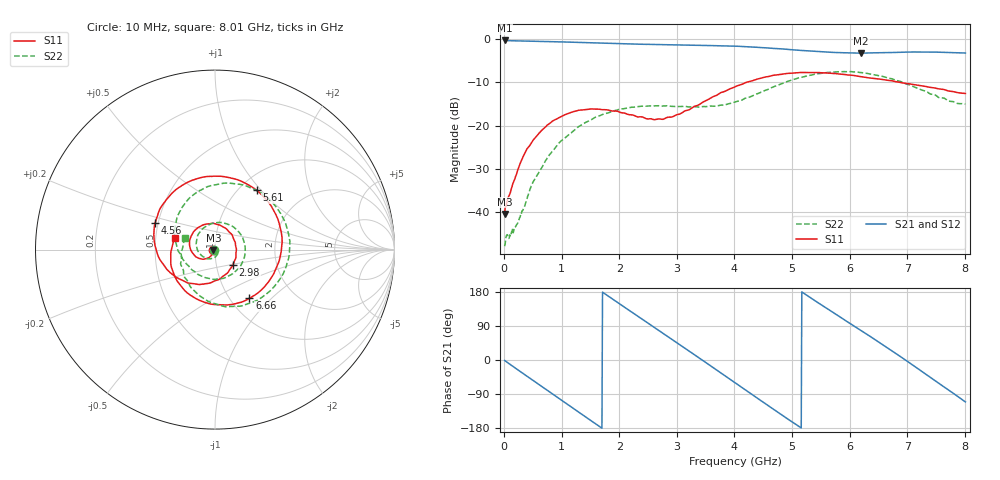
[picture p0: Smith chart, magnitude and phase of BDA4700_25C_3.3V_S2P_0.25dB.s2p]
!Agilent Technologies,E5071B,MY42404982,A.09.10
!Date: Mon Oct 20 18:03:04 2025
!Data & Calibration Information:
!Freq	S11:SOLT2(ON)	S21:SOLT2(ON)	S12:SOLT2(ON)	S22:SOLT2(ON)
# Hz S RI R 50
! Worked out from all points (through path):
!   801 points, 10 MHz to 8.01 GHz, reference 50 ohm
!   highest |S21| = -0.37 dB at 10 MHz (marker M1); lowest = -3.3 dB at 6.2 GHz (marker M2)
!   group delay of S21, straight-line fit = 286 ps
!   lowest |S11| = -40.4 dB at 10 MHz (marker M3), VSWR 1.02, Z = 49.1 - j0.238 ohm
!   |S11| at or under -10 dB: start of sweep to 4.215 GHz; 6.86 GHz to end of sweep
!   |S22| runs from -47.8 to -7.5 dB; largest |S21 - S12| = 0.011
!   S11 on the Smith chart (normalised r, x): 10 MHz: 0.98, -0.00; 2.98 GHz: 1.20, -0.21; 4.56 GHz: 0.48, +0.16; 5.61 GHz: 1.19, +0.95; 6.66 GHz: 1.22, -0.75; 8.01 GHz: 0.63, +0.09
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1e7  -0.00927 -0.00243  0.9577 -0.0205  0.9574 -0.0212  -0.00405 -0.000447
3.6e8  -0.0273 -0.0393  0.7354 -0.5892  0.735 -0.5896  0.0118 -0.000516
7.1e8  -0.0803 -0.0511  0.2291 -0.903  0.2287 -0.903  0.00503 -0.0378
1.02e9  -0.1289 -0.0133  -0.2922 -0.8734  -0.2922 -0.873  -0.0482 -0.049
1.35e9  -0.1377 0.0624  -0.7279 -0.5431  -0.7278 -0.5434  -0.1014 0.0106
1.64e9  -0.0935 0.1233  -0.89 -0.0992  -0.8904 -0.0987  -0.0859 0.0957
1.92e9  -0.021 0.1456  -0.8139 0.3439  -0.8145 0.3435  -0.00336 0.1485
2.32e9  0.0793 0.0975  -0.3781 0.7821  -0.3783 0.7821  0.1337 0.0972
2.68e9  0.1191 0.00486  0.1689 0.8426  0.168 0.8425  0.1643 -0.0414
2.98e9  0.0998 -0.0861  0.5733 0.6297  0.5724 0.6289  0.0986 -0.1343
3.48e9  -0.0337 -0.1877  0.8378 -0.063  0.8381 -0.063  -0.0666 -0.1517
4.01e9  -0.2486 -0.1294  0.4128 -0.7114  0.4143 -0.7102  -0.1786 -0.0541
4.56e9  -0.3335 0.1484  -0.3652 -0.6964  -0.3645 -0.6977  -0.2207 0.1333
4.95e9  -0.1951 0.3494  -0.6987 -0.2804  -0.6987 -0.2845  -0.1231 0.3031
5.35e9  0.0655 0.4036  -0.6825 0.2308  -0.684 0.2269  0.1153 0.3659
5.61e9  0.2317 0.3317  -0.5017 0.4912  -0.5031 0.4914  0.2797 0.2986
6.2e9  0.3645 -0.034  0.1428 0.6687  0.1522 0.6698  0.3987 -0.0867
6.66e9  0.1915 -0.2717  0.5911 0.3636  0.5924 0.3629  0.1901 -0.2998
6.68e9  0.1804 -0.278  0.6033 0.3436  0.6055 0.3421  0.1782 -0.3035
7.24e9  -0.1375 -0.2536  0.6199 -0.3387  0.6188 -0.3386  -0.111 -0.2338
7.63e9  -0.2445 -0.0917  0.2383 -0.6565  0.2379 -0.6567  -0.1914 -0.0813
8.01e9  -0.2254 0.0647  -0.2413 -0.6423  -0.2384 -0.6431  -0.1655 0.0638
